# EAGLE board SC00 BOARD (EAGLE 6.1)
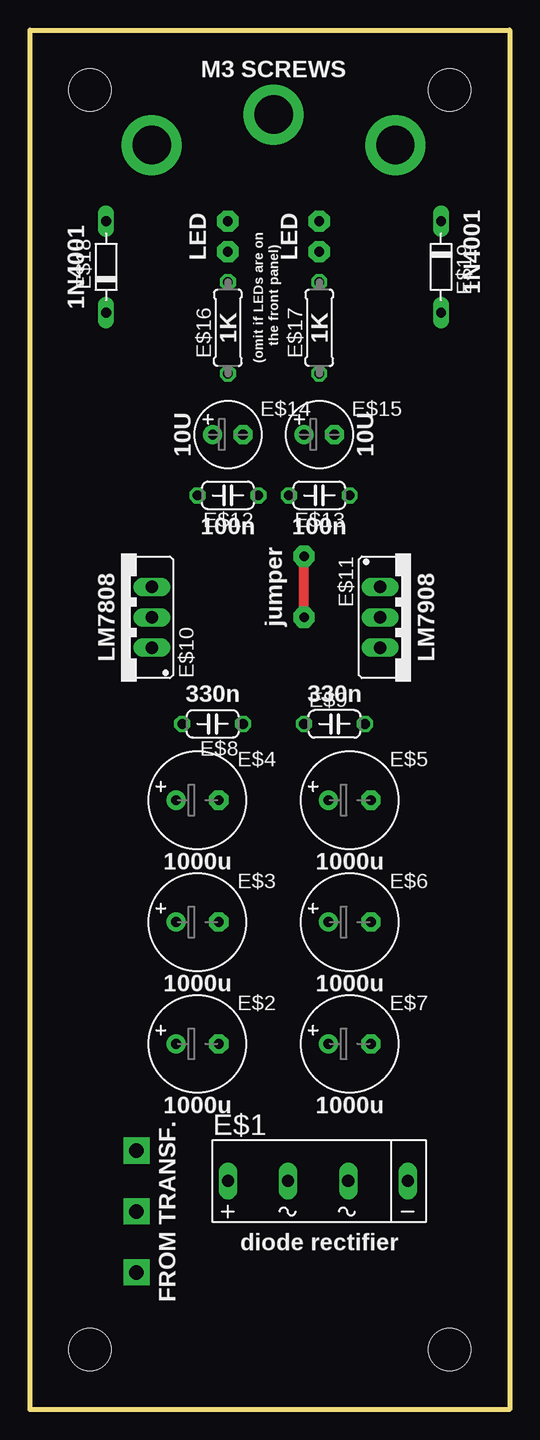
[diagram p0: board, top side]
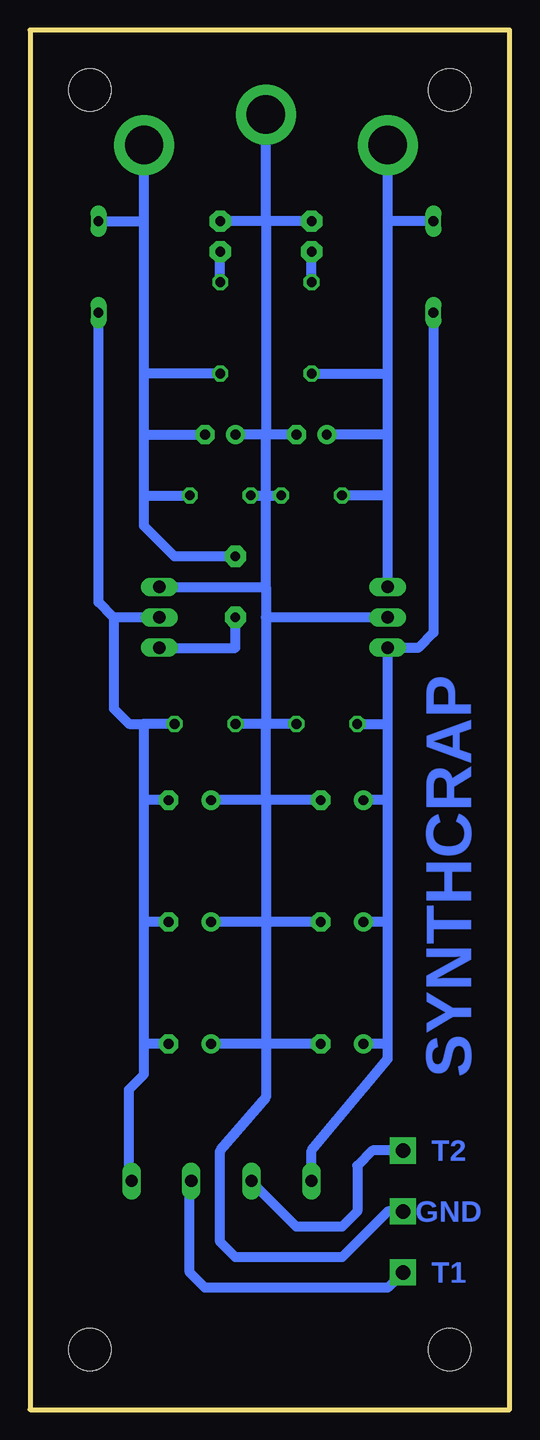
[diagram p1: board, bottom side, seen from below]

Size 40 x 115 mm. Coordinates in mm from the lower left corner, seen from the top.
Outline: 0,0 0,115 40,115 40,0 0,0
Copper layers (1*16): Top 0.035mm / dielectric 1.5mm / Bottom 0.035mm
Design rules: minimum track width 10mil, minimum drill 24mil, track to track 8mil, track to pad 8mil, pad to pad 8mil, via to via 8mil, smd to smd 8mil, copper to edge 40mil, drill to drill 8mil, minimum pad ring 10mil, minimum via ring 8mil, stop-mask expansion 4mil, vias tented up to drill 0mil, thermal gap 10mil
Holes 3.5 mm at 5,5 35,5 5,110 35,110

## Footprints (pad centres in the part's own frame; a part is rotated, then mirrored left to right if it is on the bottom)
2KBB-R = drill 1.016 long: + -7.62,0; - 7.391,0; AC1 -2.616,0; AC2 2.413,0
E3,5-8 = drill 0.813 pad 1.6: + -1.778,0 | drill 0.813 pad 1.6 octagon: - 1.778,0
C050-024X044 = drill 0.813 octagon: 1 -2.54,0; 2 2.54,0
78XXS = drill 1.016 long: GND 0,-2.54; IN -2.54,-2.54; OUT 2.54,-2.54
79XXS = drill 1.016 long: GND -2.54,-2.54; IN 0,-2.54; OUT 2.54,-2.54
E2,5-6 = drill 0.813 pad 1.6: + -1.27,0 | drill 0.813 pad 1.6 octagon: - 1.27,0
0207/7 = drill 0.813 octagon: 1 -3.81,0; 2 3.81,0
D-7.5 = drill 0.813 long: A 3.81,0; C -3.81,0

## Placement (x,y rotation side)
E$1  [2KBB-R]  24.13,19.05 0 top
E$2  [E3,5-8]  13.97,30.48 0 top
E$3  [E3,5-8]  13.97,40.64 0 top
E$4  [E3,5-8]  13.97,50.8 0 top
E$5  [E3,5-8]  26.67,50.8 0 top
E$6  [E3,5-8]  26.67,40.64 0 top
E$7  [E3,5-8]  26.67,30.48 0 top
E$8  [C050-024X044]  15.24,57.15 180 top
E$9  [C050-024X044]  25.4,57.15 0 top
E$10  [78XXS]  7.62,66.04 90 top
E$11  [79XXS]  31.75,66.04 270 top
E$12  [C050-024X044]  16.51,76.2 180 top
E$13  [C050-024X044]  24.13,76.2 180 top
E$14  [E2,5-6]  16.51,81.28 0 top
E$15  [E2,5-6]  24.13,81.28 0 top
E$16  [0207/7]  16.51,90.17 90 top
E$17  [0207/7]  24.13,90.17 90 top
E$18  [D-7.5]  6.35,95.25 90 top
E$19  [D-7.5]  34.29,95.25 270 top

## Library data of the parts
E$1 = rectifier
E$2-E$9 E$12-E$17 = rcl
E$10 E$11 = v-reg
E$18 E$19 = diode

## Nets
S$2: E$16.2
S$4: E$8.1 E$9.1 E$10.GND E$11.GND E$12.1 E$13.2 E$14.- E$15.+
S$6: E$9.2 E$11.IN E$19.A
S$7: E$1.+ E$8.2 E$10.IN E$18.C
S$9: E$17.2
S$10: E$11.OUT E$13.1 E$15.- E$17.1 E$19.C
S$11: E$10.OUT E$12.2 E$14.+ E$16.1 E$18.A

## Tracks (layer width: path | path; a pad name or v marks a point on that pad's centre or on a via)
S$2  (via drill 0.8 pad 1.78)
  Bottom 0.813: E$16.2 v16.51,96.52
S$3  (via drill 1.2 pad 2.18)
  Bottom 0.813: v8.89,11.43 10.16,10.16 25.4,10.16 26.67,11.43 26.67,19.05
S$4  (via drill 0.8 pad 1.78, 1.2 pad 2.18, 3.2 pad 5)
  Bottom 0.813: v16.51,99.06 20.32,99.06 | 20.32,99.06 v24.13,99.06 | E$11.GND 20.32,68.58 | E$10.GND 20.32,66.04 | 15.88,50.8 20.32,50.8 | 20.32,50.8 24.77,50.8 | 15.88,40.64 20.32,40.64 | 20.32,40.64 24.77,40.64 | 20.32,50.8 20.32,40.64 | 15.88,30.48 20.32,30.48 | 20.32,30.48 24.77,30.48 | 20.32,40.64 20.32,30.48 | v8.89,16.51 10.16,16.51 13.97,12.7 22.86,12.7 24.13,13.97 24.13,21.59 20.32,26.04 20.32,30.48 | E$8.1 20.32,57.15 | 20.32,57.15 E$9.1 | 20.32,50.8 20.32,57.15 | 20.32,66.04 20.32,57.15 | 20.32,68.58 20.32,66.04 | E$13.2 20.32,76.2 | 20.32,76.2 E$12.1 | 20.32,68.58 20.32,76.2 | E$14.- 20.32,81.28 | 20.32,81.28 E$15.+ | 20.32,76.2 20.32,81.28 | 20.32,99.06 20.32,81.28 | 20.32,99.06 v20.32,107.95
S$5  (via drill 1.2 pad 2.18)
  Bottom 0.813: v8.89,21.59 11.43,21.59 12.7,20.32 12.7,16.51 13.97,15.24 17.78,15.24 21.59,19.05
S$6
  Bottom 0.813: E$11.IN 33.02,66.04 | 33.02,66.04 33.02,58.42 31.75,57.15 30.48,57.15 | 31.75,19.05 31.75,26.67 30.48,27.94 30.48,30.48 | 30.48,30.48 30.48,40.64 | 30.48,40.64 30.48,50.8 | 28.57,30.48 30.48,30.48 | 28.57,40.64 30.48,40.64 | 28.57,50.8 30.48,50.8 | 30.48,50.8 30.48,57.15 | E$9.2 30.48,57.15 | 33.02,66.04 34.29,67.31 E$19.A
S$7
  Bottom 0.813: E$18.C 6.35,64.77 7.62,63.5 E$10.IN 10.16,57.15 | E$1.+ 16.51,21.59 10.16,29.21 10.16,30.48 | 10.16,30.48 10.16,40.64 | 10.16,40.64 10.16,50.8 | 10.16,50.8 12.06,50.8 | 10.16,40.64 12.06,40.64 | 10.16,30.48 12.06,30.48 | 10.16,50.8 10.16,57.15 | E$8.2 10.16,57.15
S$9  (via drill 0.8 pad 1.78)
  Bottom 0.813: E$17.2 v24.13,96.52
S$10  (via drill 0.8 pad 1.78, 3.2 pad 5)
  Top 0.813: v22.86,66.04 v22.86,71.12
  Bottom 0.813: E$11.OUT 22.86,63.5 v22.86,66.04 | v22.86,71.12 27.94,71.12 30.48,73.66 30.48,76.2 | 30.48,76.2 E$13.1 | 30.48,76.2 30.48,81.28 | 30.48,81.28 E$15.- | 30.48,81.28 30.48,86.36 | 30.48,86.36 30.48,99.06 | 30.48,99.06 v30.48,105.41 | E$17.1 30.48,86.36 | E$19.C 30.48,99.06
S$11  (via drill 3.2 pad 5)
  Bottom 0.813: E$10.OUT 10.16,76.2 | 10.16,76.2 E$12.2 | 10.16,76.2 10.16,81.28 | 10.16,81.28 E$14.+ | 10.16,81.28 10.16,86.36 | 10.16,86.36 10.16,99.06 | 10.16,99.06 v10.16,105.41 | E$16.1 10.16,86.36 | E$18.A 10.16,99.06

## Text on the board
Bottom: SYNTHCRAP | T2 | GND | T1
tPlace: M3 SCREWS | LED | LED | 1N4001 | 1N4001 | (omit if LEDs are on | the front panel) | 1K | 1K | 10U | 10U | 100n | 100n | jumper | LM7808 | LM7908 | 330n | 330n | 1000u | 1000u | 1000u | 1000u | 1000u | 1000u | FROM TRANSF. | diode rectifier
